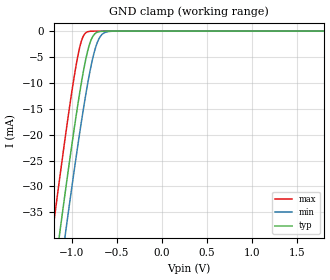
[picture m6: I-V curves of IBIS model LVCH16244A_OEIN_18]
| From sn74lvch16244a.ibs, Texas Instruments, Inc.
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[Model]   LVCH16244A_OEIN_18
Model_type  Input
Vinl=0.5775
Vinh=1.2675
| variable   typ   min   max
C_comp   3.47pF   2.69pF   4.45pF
[Temperature Range]   40   100   -40
| Ambient temperature   25   85   -40
[Voltage range]   1.8   1.65   1.95
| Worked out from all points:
|   GND clamp passes 1 mA (typ) near -0.77 V on its own axis
[GND Clamp]
| LVCH16244A_OEIN_18
|   Voltage   I(typ)   I(min)   I(max)
-5V       -583.8mA   -590.8mA   -575.1mA
-1.21V    -48.93mA   -57.22mA   -38.3mA
-1.135V   -39.07mA   -47.36mA   -28.42mA
-1.075V   -31.35mA   -39.6mA    -20.75mA
-1.06V    -29.44mA   -37.69mA   -18.89mA
-960mV    -17.26mA   -25.26mA   -7.377mA
-885mV    -9.098mA   -16.55mA   -1.486mA
-830mV    -4.281mA   -10.75mA   -171.6uA
-780mV    -1.472mA   -6.227mA   -17.15uA
-715mV    -205.4uA   -2.128mA   -808.5nA
-650mV    -22.01uA   -443.9uA   -37.93nA
1.8V      3.326pA    6.142pA    3.026pA
